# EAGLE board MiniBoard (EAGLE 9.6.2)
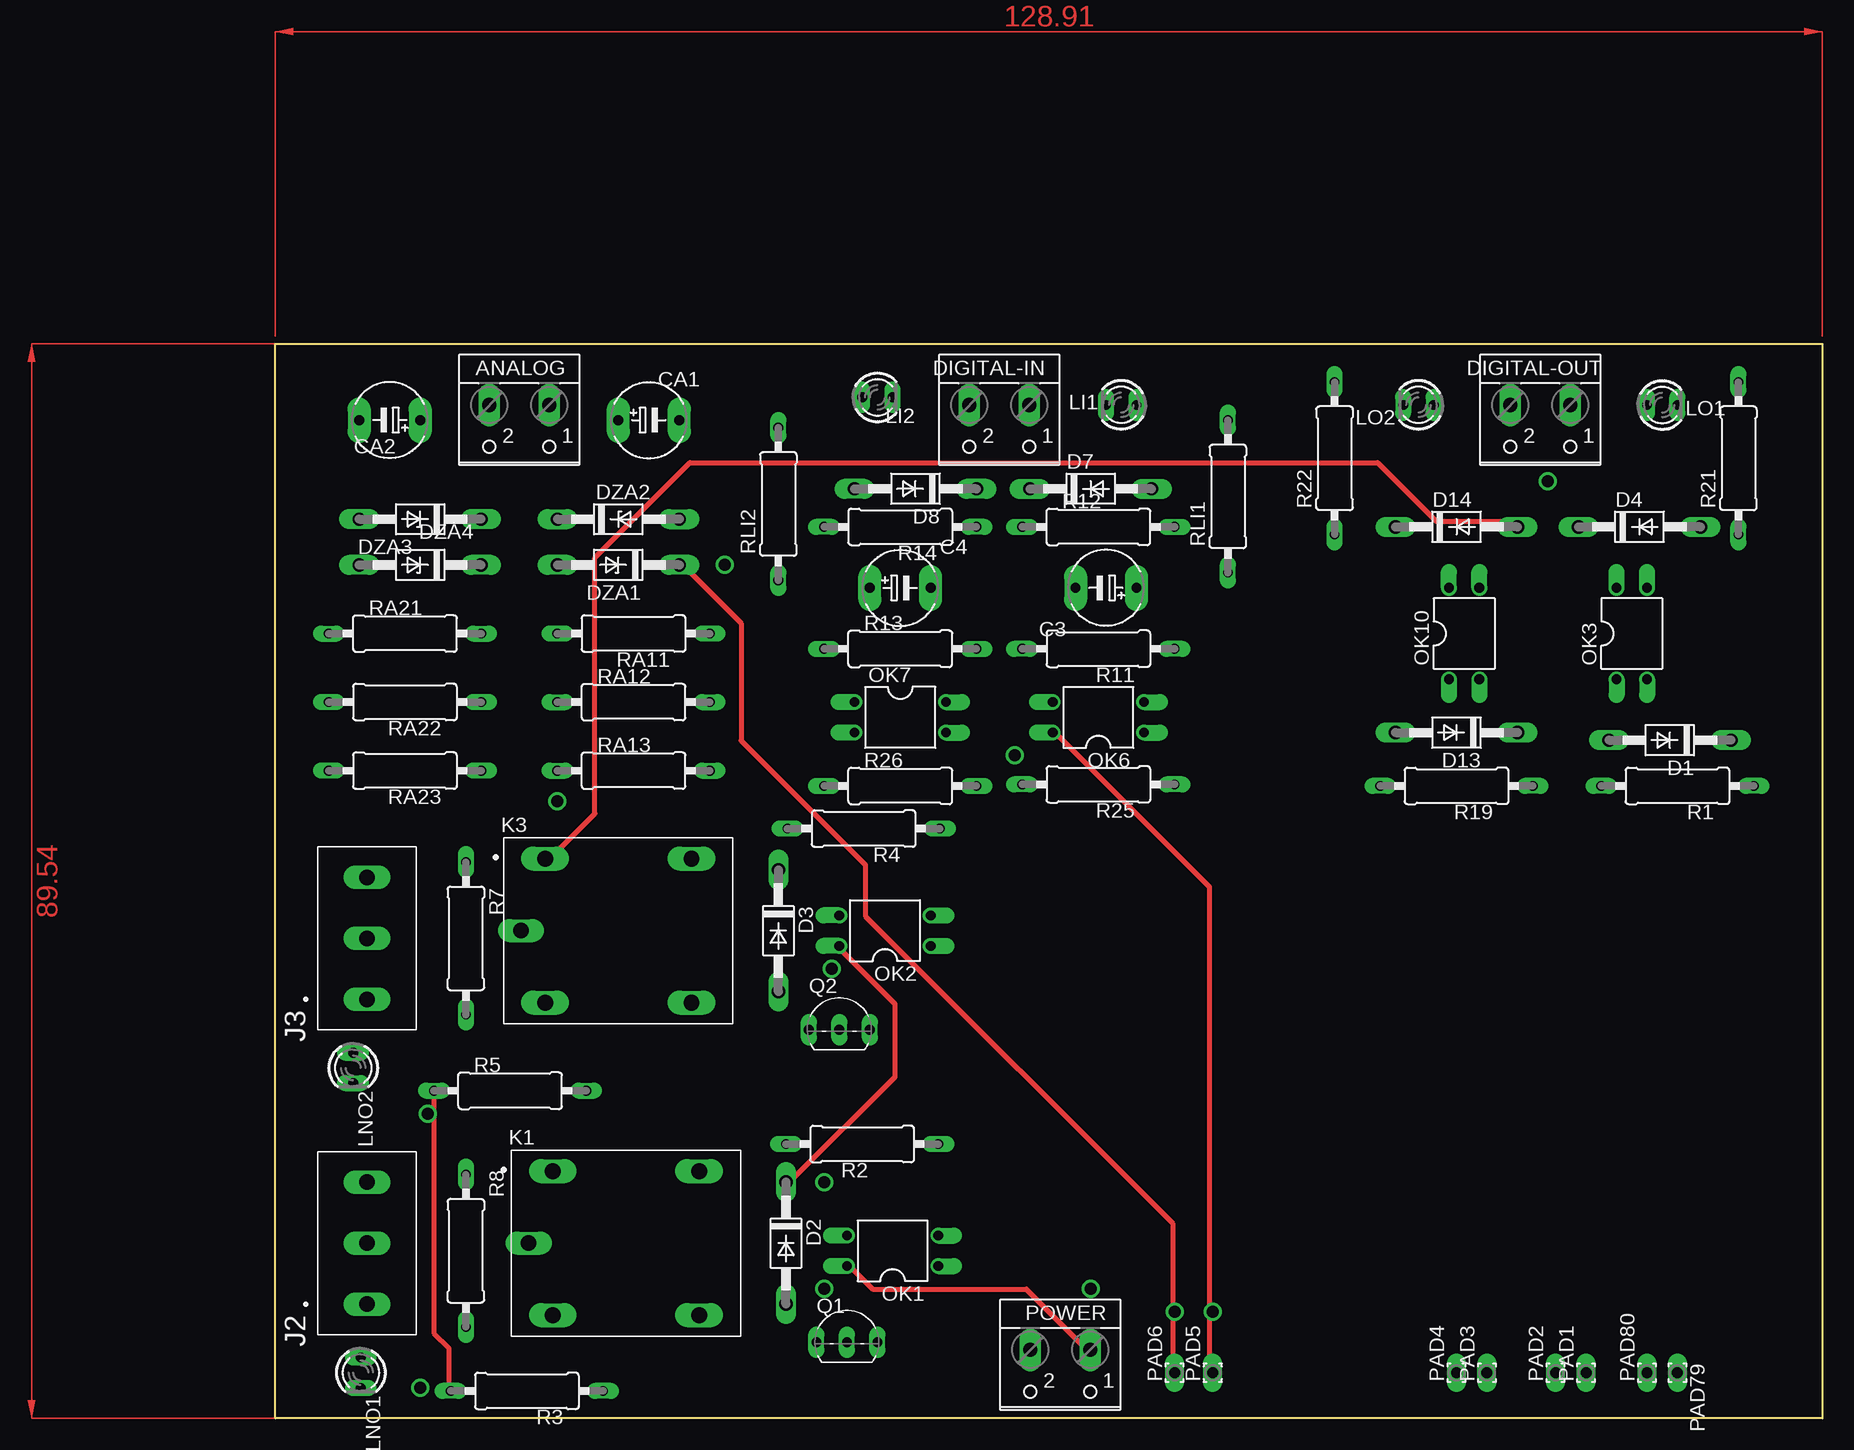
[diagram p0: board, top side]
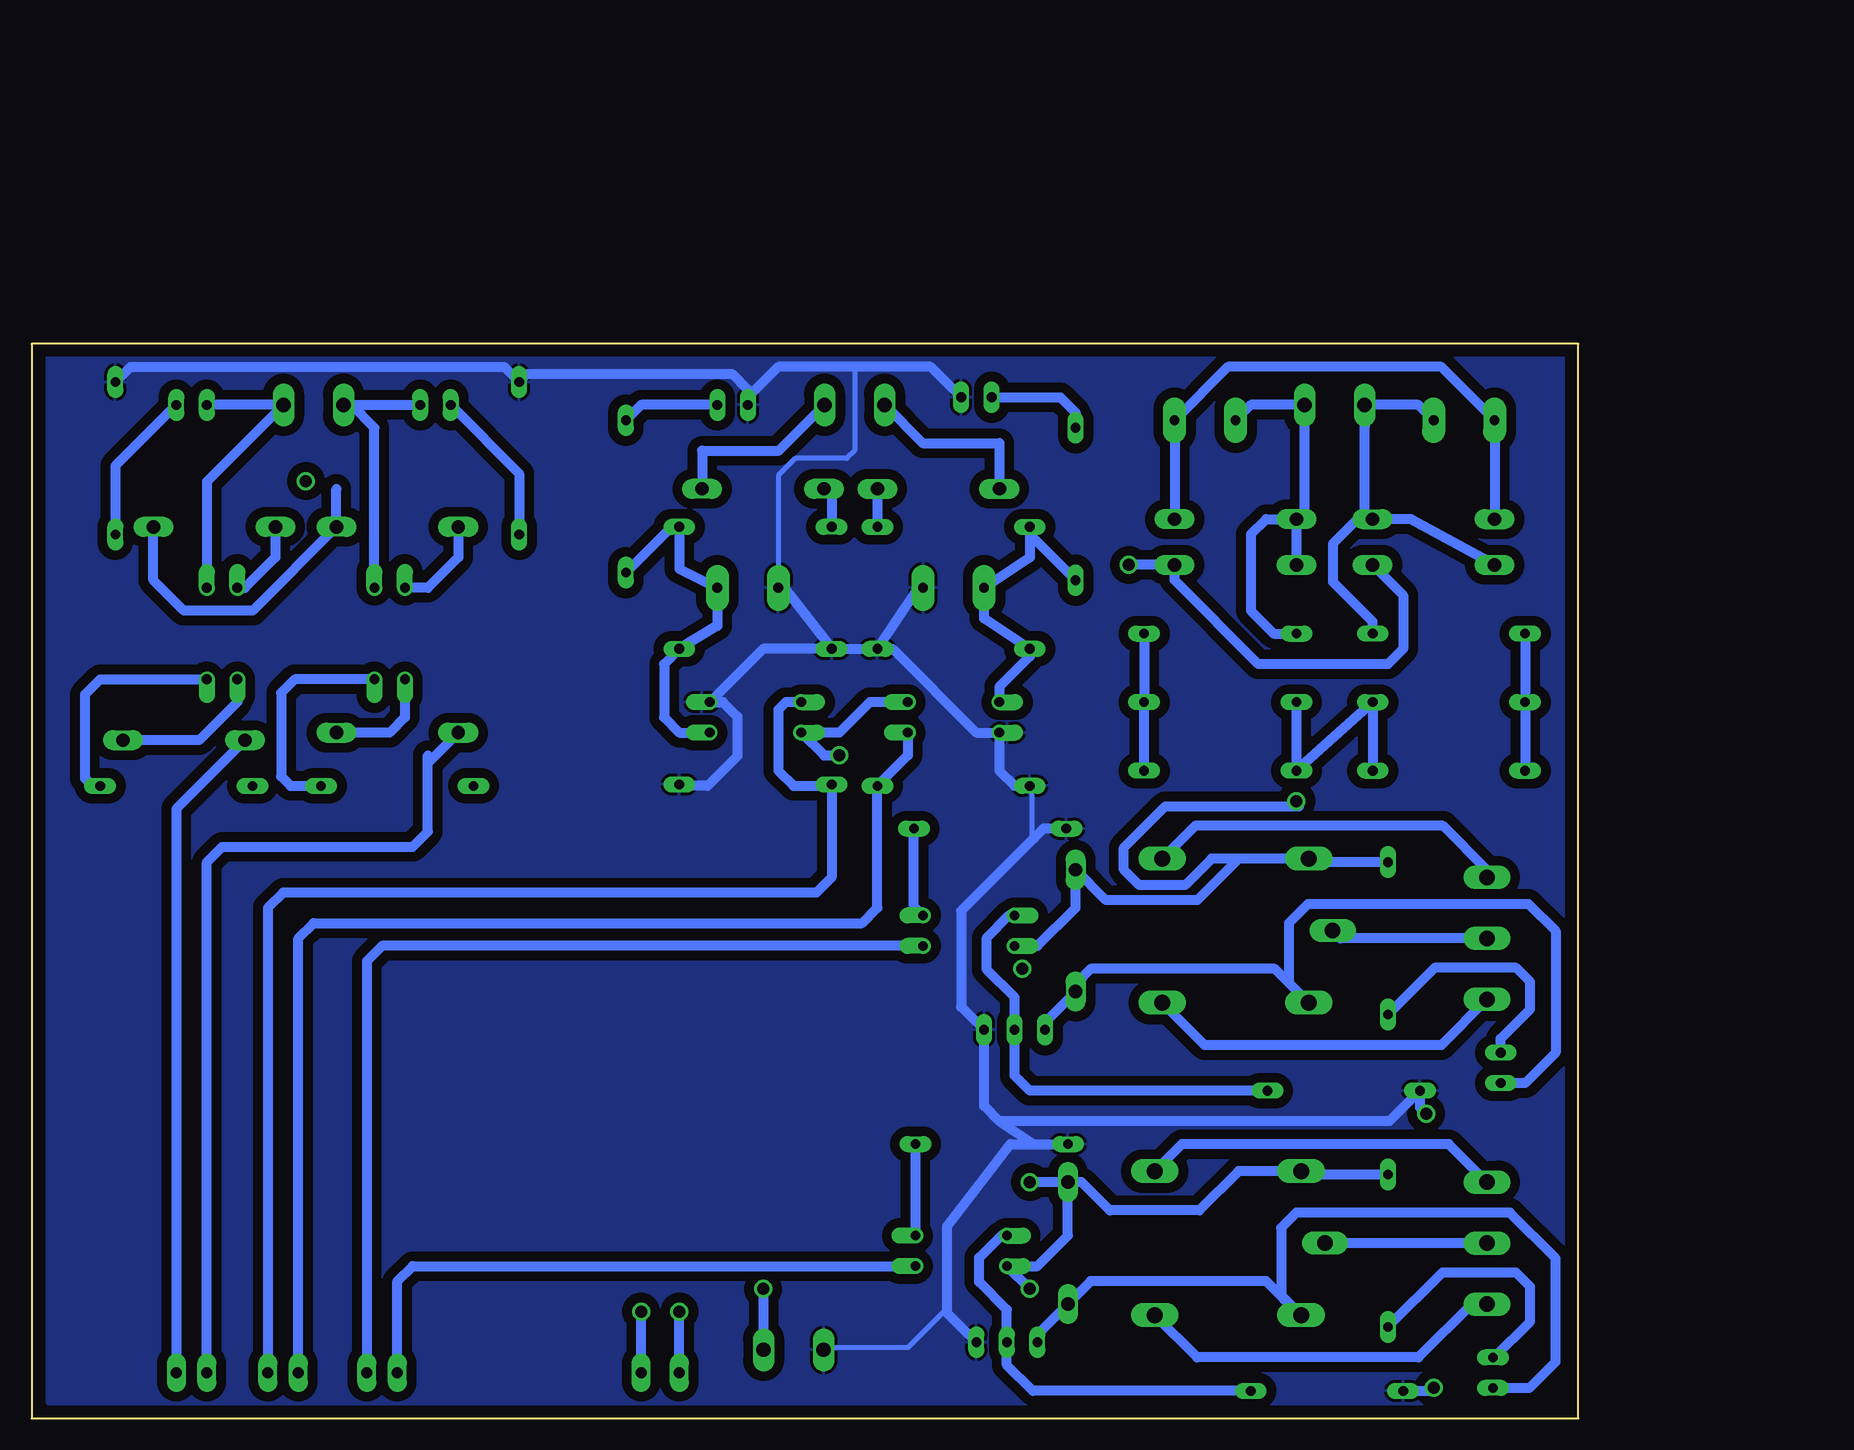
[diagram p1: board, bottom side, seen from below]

Size 128.91 x 89.54 mm. Coordinates in mm from the lower left corner, seen from the top.
Outline: 0,89.54 128.91,89.54 128.91,0 0,0 0,89.54
Copper layers (1*16): Top 0.035mm / dielectric 1.5mm / Bottom 0.035mm
Design rules "default *": minimum track width 16mil, minimum drill 0.35mm, track to track 32mil, track to pad 32mil, pad to pad 32mil, via to via 32mil, smd to smd 6mil, copper to edge 40mil, drill to drill 6mil, minimum pad ring 10mil, minimum via ring 8mil, stop-mask expansion 4mil, vias tented up to drill 0mil, thermal gap 10mil

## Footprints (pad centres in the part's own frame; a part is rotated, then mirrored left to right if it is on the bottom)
W237-102 = drill 1.194 long: 1 -2.5,-1.27; 2 2.5,-1.27
E5-6 = drill 0.813 pad 1.905 long: + -2.54,0; - 2.54,0
DO41-10 = drill 1.118 long: A 5.08,0; C -5.08,0
DO41Z10 = drill 1.118 long: A 5.08,0; C -5.08,0
CUI_TB006-508-03BE = drill 1.3 long: 1 0,0; 2 5.08,0; 3 10.16,0
RELAY_SRD-05VDC-SL-C = drill 1.32 long: A1 -6.1,6; A2 -6.1,-6; NC 6.1,6; NO 6.1,-6 | drill 1.29 long: COM -8.1,0
LED3MM = drill 0.813 long: A -1.27,0; K 1.27,0
DIL04 = drill 0.813 offset: 1 -1.27,-3.81; 2 1.27,-3.81; 3 1.27,3.81; 4 -1.27,3.81
1,6/0,9 = drill 0.914 pad 1.6 long: 1 0,0
TO92-EBC = drill 0.813 long: B 0,-1.27; C -2.54,-1.27; E 2.54,-1.27
0309/12 = drill 0.813 long: 1 -6.35,0; 2 6.35,0

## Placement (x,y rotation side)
ANALOG  [W237-102]  20.32,83.19 180 top
C3  100n  [E5-6]  69.22,69.22 180 top
C4  100n  [E5-6]  52.07,69.22 0 top
CA1  100n  [E5-6]  31.12,83.19 0 top
CA2  100n  [E5-6]  9.53,83.19 180 top
D1  1N4004  [DO41-10]  116.2,56.52 180 top
D2  1N4004  [DO41-10]  42.55,14.61 270 top
D3  1N4004  [DO41-10]  41.91,40.64 270 top
D4  1N4004  [DO41-10]  113.67,74.3 0 top
D7  1N4004  [DO41-10]  67.95,77.47 0 top
D8  1N4004  [DO41-10]  53.34,77.47 180 top
D13  1N4004  [DO41-10]  98.42,57.15 180 top
D14  1N4004  [DO41-10]  98.42,74.3 0 top
DIGITAL-IN  [W237-102]  60.33,83.19 180 top
DIGITAL-OUT  [W237-102]  105.41,83.19 180 top
DZA1  1N4728  [DO41Z10]  28.58,71.12 180 top
DZA2  1N4728  [DO41Z10]  28.58,74.93 0 top
DZA3  1N4728  [DO41Z10]  12.06,71.12 180 top
DZA4  1N4728  [DO41Z10]  12.06,74.93 180 top
J2  WAGO-03BE  [CUI_TB006-508-03BE]  7.62,9.53 90 top
J3  WAGO-03BE  [CUI_TB006-508-03BE]  7.62,34.92 90 top
K1  SRD-05VDC-SL-C  [RELAY_SRD-05VDC-SL-C]  29.21,14.61 0 top
K3  SRD-05VDC-SL-C  [RELAY_SRD-05VDC-SL-C]  28.58,40.64 0 top
LI1  [LED3MM]  70.48,84.45 180 top
LI2  [LED3MM]  50.16,85.09 0 top
LNO1  [LED3MM]  7.11,3.81 270 top
LNO2  [LED3MM]  6.48,29.21 270 top
LO1  [LED3MM]  115.57,84.45 0 top
LO2  [LED3MM]  95.25,84.45 180 top
OK1  PC817  [DIL04]  51.44,13.97 90 top
OK2  PC817  [DIL04]  50.8,40.64 90 top
OK3  PC817  [DIL04]  113.03,65.41 0 top
OK6  PC817  [DIL04]  68.58,58.42 90 top
OK7  PC817  [DIL04]  52.07,58.42 270 top
OK10  PC817  [DIL04]  99.06,65.41 0 top
PAD1  WIREPAD1,6/0,9  [1,6/0,9]  109.22,3.81 90 top
PAD2  WIREPAD1,6/0,9  [1,6/0,9]  106.68,3.81 90 top
PAD3  WIREPAD1,6/0,9  [1,6/0,9]  100.97,3.81 90 top
PAD4  WIREPAD1,6/0,9  [1,6/0,9]  98.42,3.81 90 top
PAD5  WIREPAD1,6/0,9  [1,6/0,9]  78.11,3.81 90 top
PAD6  WIREPAD1,6/0,9  [1,6/0,9]  74.93,3.81 90 top
PAD79  WIREPAD1,6/0,9  [1,6/0,9]  116.84,3.81 270 top
PAD80  WIREPAD1,6/0,9  [1,6/0,9]  114.3,3.81 90 top
POWER  [W237-102]  65.41,4.45 180 top
Q1  BC338  [TO92-EBC]  47.62,7.62 0 top
Q2  BC338  [TO92-EBC]  46.99,33.66 0 top
R1  220  [0309/12]  116.84,52.7 180 top
R2  220  [0309/12]  48.9,22.86 180 top
R3  2K  [0309/12]  20.95,2.29 180 top
R4  220  [0309/12]  49.02,49.15 180 top
R5  2K  [0309/12]  19.56,27.31 0 top
R7  2K  [0309/12]  15.87,40.01 270 top
R8  2K  [0309/12]  15.87,13.97 270 top
R11  470  [0309/12]  68.58,64.14 180 top
R12  2K  [0309/12]  68.58,74.3 0 top
R13  470  [0309/12]  52.07,64.14 0 top
R14  2K  [0309/12]  52.07,74.3 180 top
R19  220  [0309/12]  98.42,52.7 180 top
R21  [0309/12]  121.92,80.01 90 top
R22  [0309/12]  88.27,80.01 90 top
R25  180  [0309/12]  68.58,52.83 180 top
R26  180  [0309/12]  52.07,52.7 0 top
RA11  100K  [0309/12]  29.84,65.41 180 top
RA12  10K  [0309/12]  29.84,59.69 0 top
RA13  1K  [0309/12]  29.84,53.98 0 top
RA21  100K  [0309/12]  10.79,65.41 0 top
RA22  10K  [0309/12]  10.79,59.69 180 top
RA23  1K  [0309/12]  10.79,53.98 180 top
RLI1  [0309/12]  79.38,76.84 90 top
RLI2  [0309/12]  41.91,76.2 90 top

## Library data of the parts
ANALOG DIGITAL-IN DIGITAL-OUT POWER = con-wago-500; MPN: 237-102; OC_FARNELL: unknown; OC_NEWARK: 70K9898
C3 C4 CA1 CA2 = rcl-ws; SPICEPREFIX: C
D1-D4 D7 D8 D13 D14 = diode
DZA1-DZA4 = diode-ws
J2 J3 = TB006-508-03BE; AVAILABILITY: In Stock; CHECK_PRICES: https://www.snapeda.com/parts/TB006-508-03BE/Same+Sky/view-part/?ref=eda; DESCRIPTION: 2~24 Poles, Screw Type, Horizontal, 5.08 Pitch, 26~14 (AWG), Terminal Block Connector; MF: Same Sky; MP: TB006-508-03BE; PACKAGE: None; PRICE: None; SNAPEDA_LINK: https://www.snapeda.com/parts/TB006-508-03BE/Same+Sky/view-part/?ref=snap
K1 K3 = SRD-05VDC-SL-C; AVAILABILITY: In Stock; CHECK_PRICES: https://www.snapeda.com/parts/SRD-05VDC-SL-C/Songle+Relay/view-part/?ref=eda; DESCRIPTION: 5V Trigger Relay Module For Arduino And Raspberry Pi 5V Trigger Relay Module For Arduino And Raspberry Pi; MF: Songle Relay; MP: SRD-05VDC-SL-C; PACKAGE: NON STANDARD-5 Songle Relay; PRICE: None; SNAPEDA_LINK: https://www.snapeda.com/parts/SRD-05VDC-SL-C/Songle+Relay/view-part/?ref=snap
LI1 LI2 LNO1 LNO2 LO1 LO2 = led_WS
OK1-OK3 OK6 OK7 OK10 = optocoupler; MPN: PC817X4J000F; OC_FARNELL: 9707727; OC_NEWARK: 97K7059
PAD1-PAD6 PAD79 PAD80 = wirepad-ws
Q1 Q2 = transistor-npn
R1-R5 R7 R8 R11-R14 R19 R21 R22 R25 R26 RA11-RA13 RA21-RA23 RLI1 RLI2 = rcl-ws; SPICEPREFIX: R

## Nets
3V3: OK6.4 OK7.4 PAD5.1
5V: DZA1.C DZA3.C PAD6.1
12V: D2.C D3.C D4.A D14.A K1.A1 K3.A1 OK1.4 OK2.4 POWER.1 R7.1 R8.1
A1: RA11.1 RA12.2 RA13.2
A2: RA21.1 RA22.2 RA23.2
AI1: ANALOG.1 CA1.+ DZA1.A DZA2.C RA11.2
AI2: ANALOG.2 CA2.+ DZA3.A DZA4.C RA21.2
COM1: J2.2 K1.COM
COM2: J3.2 K3.COM
GND: C3.- C4.- LI1.K LI2.K OK6.2 OK7.2 POWER.2 Q1.E Q2.E R2.2 R3.2 R4.2 R5.1 R11.2 R13.2 R21.2 R22.2 R25.1 R26.1
IN1: D7.A DIGITAL-IN.1
IN2: D8.A DIGITAL-IN.2
N$1: OK2.2 R4.1
N$2: OK1.2 R2.1
N$3: OK1.3 Q1.B R3.1
N$4: D3.A K3.A2 LNO2.K Q2.C
N$6: OK2.3 Q2.B R5.2
N$7: LNO2.A R7.2
N$10: LNO1.A R8.2
N$11: D2.A K1.A2 LNO1.K Q1.C
N$15: D1.C OK3.1
N$16: OK3.2 R1.1
N$18: D4.C OK3.4
N$19: C3.+ OK6.1 R11.1 R12.2 RLI1.1
N$20: D7.C R12.1
N$21: C4.+ OK7.1 R13.1 R14.2 RLI2.1
N$22: D8.C R14.1
N$24: LI2.A RLI2.2
N$26: D13.C OK10.1
N$27: OK10.2 R19.1
N$29: LI1.A RLI1.2
N$30: LO1.K R21.1
N$31: LO2.K R22.1
N$34: RA12.1 RA13.1 RA22.1 RA23.1
N$35: CA1.- CA2.- DZA2.A DZA4.A
N$52: D14.C OK10.4
NC1: J2.3 K1.NC
NC2: J3.3 K3.NC
NO1: J2.1 K1.NO
NO2: J3.1 K3.NO
OUT1: DIGITAL-OUT.1 LO1.A OK3.3
OUT2: DIGITAL-OUT.2 LO2.A OK10.3
R1: D1.A PAD79.1
R2: D13.A PAD80.1
RR1: OK1.1 PAD4.1
RR2: OK2.1 PAD3.1
S1: OK6.3 PAD1.1 R25.2
S2: OK7.3 PAD2.1 R26.2

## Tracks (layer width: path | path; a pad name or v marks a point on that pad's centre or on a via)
3V3
  Top 0.406: PAD5.1 77.83,4.06 77.83,44.3 65.02,57.1 OK6.4
  Bottom 0.813: OK7.4 59.06,59.69 61.59,57.15 OK6.4 62.86,55.25 61.59,55.25 | PAD5.1 78.11,8.89
5V
  Top 0.406: PAD6.1 74.78,4.06 74.78,16.26 49.17,41.86 49.17,46.13 38.81,56.49 38.81,66.24 33.93,71.12 DZA1.C
  Bottom 0.813: DZA3.C 14.6,68.58 14.6,64.14 15.87,62.87 26.67,62.87 33.66,69.85 DZA1.C 37.47,71.12 | PAD6.1 74.93,8.89
12V  (via drill 0.35)
  Top 0.406: POWER.1 67.46,5.89 62.59,10.77 49.78,10.77 47.95,12.6 OK1.4 | D14.A 103.43,74.78 96.72,74.78 91.85,79.65 34.54,79.65 26.62,71.73 26.62,50.39 22.96,46.74 K3.A1 | D2.C 43.08,19.91 51.61,28.45 51.61,34.54 47.35,38.81 OK2.4
  Bottom 0.813: R7.1 22.19,46.36 K3.A1 | K3.A1 28.29,46.64 31.75,43.18 39.37,43.18 D3.C 41.91,42.55 45.09,39.37 OK2.4 | R8.1 22.83,20.32 K1.A1 28.31,20.61 31.58,17.33 39.04,17.33 41.39,19.69 D2.C | D2.C 42.55,15.24 45.09,12.7 OK1.4 45.72,10.8 | D4.A 118.75,69.85 116.2,67.31 110.49,67.31 D14.A 103.5,77.47 | 23.29,51 34.43,51 37.87,47.56 37.87,45.73 36.58,44.43 32.77,44.43 30.56,46.64 K3.A1 | POWER.1 67.91,10.76 67.95,10.8 | D2.C 45.72,19.69
  other vias: 46.99,39.37
A1
  Bottom 0.813: RA11.1 RA12.2 RA13.2
A2
  Bottom 0.813: RA21.1 RA22.2 RA23.2
AI1
  Bottom 0.813: DZA2.C 26.03,74.93 27.3,73.66 27.3,67.31 25.4,65.41 RA11.2 | CA1.+ 27.3,84.45 ANALOG.1 22.82,75.61 DZA2.C | DZA2.C DZA1.A
AI2
  Bottom 0.813: ANALOG.2 17.82,82.59 | DZA3.A 13.97,74.93 DZA4.C | RA21.2 17.15,66.39 20.47,69.72 20.47,72.87 18.41,74.93 DZA4.C | ANALOG.2 17.82,75.61 DZA4.C | CA2.+ 13.33,84.45 ANALOG.2
COM1
  Bottom 0.813: J2.2 K1.COM
COM2
  Bottom 0.813: J3.2 19.84,40.01 K3.COM
GND
  Top 0.406: R5.1 13.21,7.11 14.43,5.89 14.43,2.85 R3.2
  Bottom 0.406: 60.33,87.63 60.33,80.64 60.96,80.01 65.26,80.01 66.67,78.59 C3.- | POWER.2 62.59,5.89 55.88,5.89 52.83,8.94 52.63,8.94 | R26.1 45.52,52.22 45.52,48.56 45.34,48.39
  Bottom 0.813: R11.2 R13.2 | R25.1 75.06,52.7 72.56,52.7 70.08,55.19 70.08,58.48 71.29,59.69 OK6.2 67.95,64.14 R11.2 | Q1.E 52.63,8.81 52.63,8.94 52.63,15.95 47.33,22.86 R2.2 45.4,22.86 48.26,24.77 | R4.2 44.58,49.15 45.34,48.39 51.44,42.29 51.44,34.29 Q2.E 49.53,26.03 48.26,24.77 | 48.26,24.77 15.75,24.77 R5.1 13.21,25.91 12.7,25.4 | C4.- 55.2,68.97 R13.2 | C3.- 66.06,69.06 R11.2 | R13.2 57.15,64.14 50.16,57.15 OK7.2 48.26,53.98 46.99,52.7 R26.1 | LI2.K 53.98,87.63 60.33,87.63 66.67,87.63 69.22,85.09 LI1.K 69.22,85.73 70.48,86.99 87.63,86.99 R22.2 89.53,87.63 120.65,87.63 R21.2 | R3.2 12.32,2.29 12.06,2.54
  pour Bottom: 1.27,89.54 127,89.54 128.27,88.27 128.27,1.91 127,0.64 1.91,0.64 0,2.54 0,3.81 0,88.27
IN1
  Bottom 0.813: DIGITAL-IN.1 66.64,80.64 73.03,80.64 D7.A
IN2
  Bottom 0.813: DIGITAL-IN.2 54.65,81.28 48.26,81.28 D8.A
N$1
  Bottom 0.813: OK2.2 55.37,42.67 R4.1
N$2
  Bottom 0.813: R2.1 OK1.2
N$3
  Bottom 0.813: R3.1 45.47,2.29 47.62,4.45 Q1.B 47.62,9.06 49.94,11.37 49.94,13.39 48.09,15.24 OK1.3
N$4
  Bottom 0.813: K3.A2 24.13,36.3 | 24.13,36.3 24.13,41.28 22.52,42.88 4.17,42.88 1.91,40.62 1.91,30.48 4.45,27.94 LNO2.K | 24.13,36.3 25.3,37.47 40.64,37.47 41.91,36.2 D3.A 44.45,33.02 Q2.C
N$5  (via drill 1 pad 0.85)
  other vias: 78.11,8.89
N$6
  Bottom 0.813: R5.2 45.72,27.31 46.99,28.58 Q2.B 46.99,35.09 49.3,37.41 49.3,40.06 47.46,41.91 OK2.3
N$7
  Bottom 0.813: LNO2.A 6.48,31.64 4.02,34.1 4.02,36.39 5.19,37.55 11.98,37.55 R7.2
N$8  (via drill 1 pad 0.85)
  other vias: 74.93,8.89
N$9  (via drill 1 pad 0.85)
  other vias: 67.95,10.8
N$10
  Bottom 0.813: LNO1.A 7,5.08 4.02,8.07 4.02,10.98 5.19,12.15 11.34,12.15 R8.2
N$11
  Bottom 0.813: LNO1.K 4.12,2.54 4.1,2.52 1.91,4.72 1.91,13.34 5.71,17.14 23.49,17.14 24.77,15.88 24.77,10.26 K1.A2 23.21,8.61 26.03,11.43 40.64,11.43 D2.A 45.09,6.98 Q1.C
N$12  (via drill 1 pad 0.85)
  other vias: 45.72,10.8
N$13  (via drill 1 pad 0.85)
  other vias: 12.06,2.54
N$14  (via drill 1 pad 0.85)
  other vias: 12.7,25.4
N$15
  Bottom 0.813: OK3.1 111.76,59.69 114.94,56.52 D1.C
N$16
  Bottom 0.813: R1.1 123.83,52.7 124.46,53.34 124.46,60.33 123.19,61.59 OK3.2
N$17  (via drill 1 pad 0.85)
  other vias: 23.49,51.44
N$18
  Bottom 0.813: OK3.4 111.12,69.22 108.59,71.76 D4.C
N$19
  Bottom 0.813: RLI1.1 75.56,74.3 R12.2 74.93,70.8 C3.+ 71.75,66.04 R11.1 76.2,62.87 76.2,58.42 74.93,57.15 OK6.1
N$20
  Bottom 0.813: D7.C 62.23,76.84 R12.1
N$21
  Bottom 0.813: RLI2.1 45.72,73.66 R14.2 45.72,71.76 C4.+ 49.53,66.67 R13.1 45.72,63.5 48.26,60.96 OK7.1
N$22
  Bottom 0.813: D8.C R14.1
N$23  (via drill 1 pad 0.85)
  other vias: 106.05,78.11
N$24
  Bottom 0.813: LI2.A 43.18,85.09 41.91,83.82 RLI2.2
N$25  (via drill 1 pad 0.85)
  other vias: 37.47,71.12
N$26
  Bottom 0.813: OK10.1 97.79,58.42 99.06,57.15 D13.C
N$27
  Bottom 0.813: OK10.2 106.97,61.59 108.1,60.46 108.1,53.49 107.31,52.7 R19.1
N$28  (via drill 1 pad 0.85)
  other vias: 61.59,55.25
N$29
  Bottom 0.813: LI1.A 78.11,84.45 RLI1.2
N$30
  Bottom 0.813: LO1.K 121.92,79.38 R21.1
N$31
  Bottom 0.813: LO2.K 88.27,78.74 R22.1
N$32  (via drill 1 pad 0.85)
  other vias: 45.72,19.69
N$33  (via drill 1 pad 0.85)
  other vias: 46.36,37.47
N$34
  Bottom 0.813: RA12.1 RA13.1 RA22.1 RA23.1
N$35
  Bottom 0.813: CA1.- 33.98,83.19 | CA1.- DZA2.A | CA1.- 29.21,87.63 11.43,87.63 CA2.- DZA4.A
N$52
  Bottom 0.813: D14.C 93.34,71.76 95.89,69.22 OK10.4
NC1
  Bottom 0.813: K1.NC 33.05,22.86 10.79,22.86 J2.3
NC2
  Bottom 0.813: J3.3 7.62,45.72 11.28,49.38 31.94,49.38 K3.NC
NO1
  Bottom 0.813: J2.1 8.89,9.53 13.33,5.08 31.79,5.08 K1.NO
NO2
  Bottom 0.813: K3.NO 31.15,31.12 11.43,31.12 J3.1
OUT1
  Bottom 0.813: OK3.3 114.3,78.07 DIGITAL-OUT.1 LO1.A
OUT2
  Bottom 0.813: OK10.3 100.33,82.55 102.23,84.45 DIGITAL-OUT.2 LO2.A
R1
  Bottom 0.813: D1.A 116.84,50.8 PAD79.1
R2
  Bottom 0.813: PAD80.1 114.3,46.36 113.03,47.62 97.16,47.62 95.89,48.89 95.89,54.61 | 95.89,54.61 95.89,55.25 | 95.89,54.61 D13.A
RR1
  Bottom 0.813: PAD4.1 98.42,11.43 97.16,12.7 OK1.1
RR2
  Bottom 0.813: OK2.1 99.7,39.37 100.97,38.1 PAD3.1
S1
  Bottom 0.813: R25.2 62.1,52.83 | OK6.3 66.04,59.69 66.67,59.06 66.67,53.98 65.41,52.7 62.36,52.7 R25.2 | PAD1.1 109.22,42.55 107.95,43.81 63.5,43.81 62.23,45.09 R25.2
S2
  Bottom 0.813: OK7.3 55.88,55.25 R26.2 58.42,42.55 59.69,41.28 105.41,41.28 106.68,40.01 PAD2.1
(copper drawn outside any net)
  shapes: Top area x2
